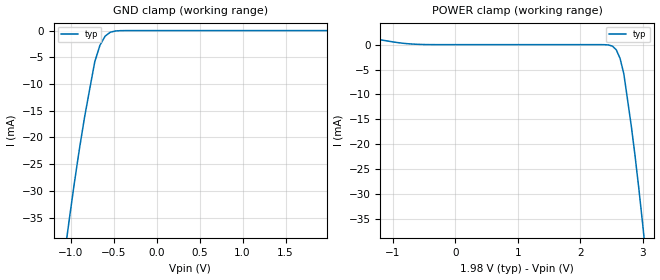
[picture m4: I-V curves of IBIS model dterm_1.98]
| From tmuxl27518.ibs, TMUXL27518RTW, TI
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| dterm_1.98
[Model]   dterm_1.98
Model_type   Terminator
|   typ   min   max
C_comp   4.014581e-12   NA   NA
[Voltage Range]   1.98   NA   NA
[Temperature Range]   27   NA   NA
[Power Clamp Reference]   1.98   NA   NA
[GND Clamp Reference]   0   NA   NA
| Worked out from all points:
|   GND clamp passes 1 mA (typ) near -0.60 V on its own axis
|   POWER clamp passes 1 mA (typ) near -1.21 V on its own axis
[GND Clamp]
|   Voltage   I(typ)   I(min)   I(max)
-3.96V    -13.08kA   NA         NA
-1.08V    -43.01mA   NA         NA
-1.02V    -35.71mA   NA         NA
-960mV    -28.77mA   NA         NA
-900mV    -22.26mA   NA         NA
-840mV    -16.31mA   NA         NA
-720mV    -5.82mA    NA         NA
-660mV    -2.757mA   NA         NA
-600mV    -1.043mA   NA         NA
-540mV    -312.1uA   NA         NA
-420mV    -15.78uA   NA         NA
1.98V     315.8pA    NA         NA
[POWER Clamp]
|   Voltage   I(typ)   I(min)   I(max)
-1.98V    2.931mA    NA         NA
-660mV    98.09uA    NA         NA
2.34V     -2.721uA   NA         NA
2.52V     -312.1uA   NA         NA
2.58V     -1.043mA   NA         NA
2.64V     -2.757mA   NA         NA
2.7V      -5.82mA    NA         NA
2.82V     -16.31mA   NA         NA
2.88V     -22.26mA   NA         NA
3V        -35.71mA   NA         NA
3.06V     -43.01mA   NA         NA
3.96V     -171.8mA   NA         NA
